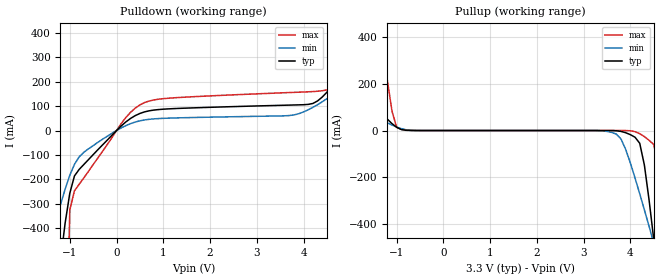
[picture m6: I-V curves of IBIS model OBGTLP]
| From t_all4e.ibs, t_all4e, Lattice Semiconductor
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|   OBGTLP
[Model]   OBGTLP
Model_type   Output
Polarity   Non-Inverting
C_comp   2pF   2pF   2pF
[Temperature Range]   25.0000   125.0000   -40.0000
[Voltage Range]   3.3000V   3.0000V   3.6000V
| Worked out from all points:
|   slope of the pulldown table from 0 to 0.495 V, typ, clamps not added: 7.1 ohm
[Pulldown]
|voltage   I(typ)   I(min)   I(max)
-3.3V     -4.47A     -1.834A    -40.58A
-1.4V     -886.8mA   -441.4mA   -5.965A
-1.1V     -380.4mA   -240.9mA   -1.121A
-900mV    -186.4mA   -138.8mA   -247.4mA
600mV     76.57mA    43.51mA    114.8mA
3.9V      105.4mA    69.14mA    157.4mA
4.6V      180.2mA    144.1mA    175.9mA
4.8V      230.4mA    173.5mA    379mA
4.9V      257.2mA    189.3mA    531.5mA
5.5V      436.8mA    293.7mA    1.547A
6.2V      665.4mA    427.9mA    2.791A
6.6V      799.6mA    508mA      3.512A
[Pullup]
|voltage   I(typ)   I(min)   I(max)
-3.3V     671.4mA    375.4mA    3.864A
-2.6V     443.5mA    240.2mA    2.608A
-1.4V     95.04mA    54.58mA    527.5mA
-1.1V     29.44mA    23.32mA    82.92mA
-900mV    4.209mA    7.979mA    4.915mA
3.6V      -117.4uA   -7.964mA   -10.28nA
4.1V      -28.73mA   -203.1mA   -4.991mA
4.3V      -148.1mA   -339.4mA   -26.09mA
4.5V      -464.6mA   -480.7mA   -59.99mA
4.6V      -640.3mA   -552.3mA   -145.8mA
4.7V      -820.2mA   -624.4mA   -980.9mA
6.6V      -4.405A    -2.027A    -34.94A
[Ramp]
| variable   typ   min   max
dV/dt_r   1.7579/2.2014ns   1.3791/2.9389ns   2.0184/1.7380ns
dV/dt_f   1.7579/1.5921ns   1.3791/3.7518ns   2.0184/0.7250ns
